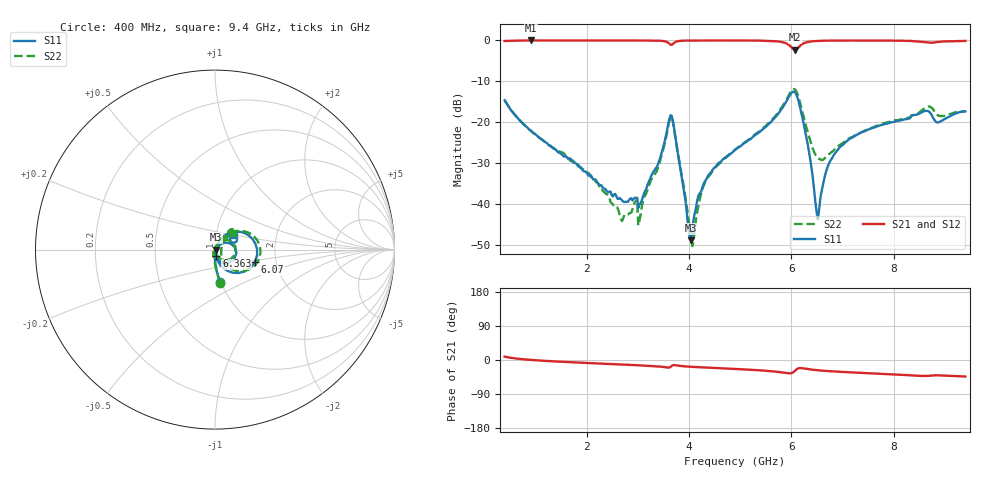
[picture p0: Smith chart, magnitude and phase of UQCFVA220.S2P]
!  Part Number UQCFVA220  Mounting Orientation: Horizontal
!  Description: Ultra Low ESR Microwave capacitors
!  Application: Coupling, Bypass, Tuning, DC Block
!  Filters, Matching
# GHZ S DB R 50
! Freq  |S11|  S11 Ph  |S21|  S21 Ph  |S12|  S12 Ph  |S22|  S22 Ph
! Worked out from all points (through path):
!   401 points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, 400 MHz to 9.4 GHz, reference 50 ohm
!   highest |S21| = 0.00 dB at 918 MHz (marker M1); lowest = -2.3 dB at 6.07 GHz (marker M2)
!   group delay of S21, straight-line fit = 14.2 ps
!   lowest |S11| = -48.9 dB at 4.045 GHz (marker M3), VSWR 1.01, Z = 50.4 + j0.0469 ohm
!   |S11| at or under -10 dB: start of sweep to end of sweep
!   |S22| runs from -50.4 to -11.9 dB; largest |S21 - S12| = 0.0036
!   S11 on the Smith chart (normalised r, x): 400 MHz: 0.99, -0.38; 6.07 GHz: 1.55, -0.23; 6.363 GHz: 1.01, -0.07; 9.4 GHz: 1.23, +0.20
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0.4  -14.64 -81.0  -0.13 8.8  -0.13 8.8  -14.63 -81.1
0.918  -22.13 -88.8  0.00 0.2  -0.01 0.2  -22.17 -90.8
1.908  -31.33 -88.2  -0.01 -7.2  -0.01 -7.3  -31.41 -105.9
2.695  -39.18 -34.6  -0.01 -12.0  -0.03 -12.1  -44.16 -170.4
2.943  -38.49 3.6  -0.01 -13.5  -0.02 -13.5  -39.58 143.7
3.055  -39.81 25.7  0.00 -14.2  -0.01 -14.2  -42.69 96.8
3.415  -29.64 43.6  -0.07 -17.1  -0.08 -17.1  -30.34 66.3
3.663  -18.43 -28.5  -1.08 -15.8  -1.07 -15.8  -18.72 -12.5
4  -47.15 -42.7  -0.03 -17.5  -0.04 -17.6  -44.25 -51.5
4.045  -48.92 7.5  -0.04 -17.9  -0.04 -17.9  -49.07 -22.5
4.315  -34.46 59.2  -0.02 -19.7  -0.03 -19.8  -34.66 68.3
4.9  -26.82 62.1  0.00 -23.6  -0.01 -23.6  -26.72 60.0
5.868  -15.68 37.3  -0.56 -33.7  -0.56 -33.7  -15.31 37.5
6.07  -12.66 -17.8  -2.28 -28.6  -2.27 -28.6  -11.99 -11.6
6.363  -28.54 -78.1  -0.28 -24.7  -0.29 -24.7  -24.28 -49.6
6.408  -32.38 -77.3  -0.21 -25.5  -0.22 -25.5  -26.11 -43.8
6.52  -43.74 4.1  -0.12 -27.1  -0.12 -27.1  -28.81 -18.8
6.7  -31.26 62.9  -0.05 -29.0  -0.06 -29.1  -28.24 15.6
6.925  -26.48 64.8  -0.03 -30.9  -0.03 -31.0  -25.73 33.1
7.915  -20.17 51.7  -0.04 -37.6  -0.05 -37.6  -19.92 43.6
8.68  -17.34 25.1  -0.53 -41.9  -0.53 -41.8  -16.17 43.5
9.4  -17.37 36.7  -0.12 -43.6  -0.14 -43.7  -17.34 44.0
